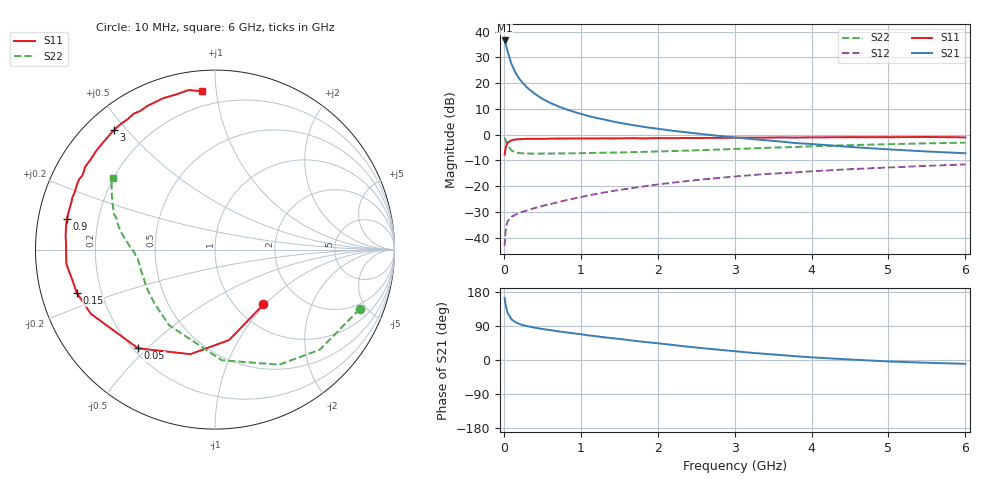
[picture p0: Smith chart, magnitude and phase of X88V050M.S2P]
! SIEMENS Small Signal Semiconductors
! BFP136W
! Si NPN RF Bipolar Junction Transistor in SOT343
! VCE = 8 V  IC = 50 mA
! Common Emitter S-Parameters:  September  1994
# GHz  S  MA  R  50
!  f  S11  S21  S12  S22
! GHz  MAG  ANG  MAG  ANG  MAG  ANG  MAG  ANG
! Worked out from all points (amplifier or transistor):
!   40 points, 10 MHz to 6 GHz, reference 50 ohm
!   highest |S21| = 36.6 dB at 10 MHz (marker M1)
!   |S21| within 3 dB of that: start of sweep to 38.22 MHz
!   unconditionally stable (mu >= 1): 786.2 MHz to 2.952 GHz
!   at 200 MHz: K = 0.52, MSG = 26.1 dB, |S12| = -30.4 dB
!   at 1.5 GHz: K = 1.11, MAG = 11.1 dB, |S12| = -21.5 dB
!   at 6 GHz: K = 0.96, MSG = 2.2 dB, |S12| = -11.6 dB
!   S11 on the Smith chart (normalised r, x): 10 MHz: 1.33, -0.98; 50 MHz: 0.22, -0.47; 150 MHz: 0.11, -0.15; 900 MHz: 0.09, +0.10; 3 GHz: 0.08, +0.46; 6 GHz: 0.11, +0.91
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0.01  0.4077 -48.5  67.69 163.9  0.0068 72.5  0.8718 -22.3
0.02  0.5099 -81.1  60.83 149.9  0.012 61.3  0.8076 -43.6
0.03  0.5984 -103.2  53.79 139.0  0.0162 53.5  0.7343 -60.8
0.05  0.6972 -127.9  40.62 124.1  0.0209 42.1  0.6177 -86.5
0.1  0.7786 -152.6  23.51 107.4  0.0253 33.9  0.4929 -121.3
0.15  0.8069 -162.6  16.19 99.8  0.0278 33.6  0.4521 -137.9
0.2  0.8126 -168.0  12.24 95.3  0.0301 33.4  0.4388 -147.4
0.25  0.8238 -172.0  9.888 92.0  0.0319 35.1  0.4332 -153.4
0.3  0.8316 -174.5  8.285 89.5  0.0336 36.7  0.4286 -157.6
0.4  0.8298 -179.2  6.249 85.3  0.0374 40.0  0.4279 -163.1
0.5  0.831 177.4  4.988 81.8  0.0411 42.4  0.4284 -166.7
0.6  0.8356 175.0  4.163 79.0  0.0446 44.5  0.4294 -169.0
0.7  0.8385 172.1  3.586 75.8  0.0484 47.2  0.4312 -170.6
0.9  0.8418 168.3  2.808 70.5  0.0567 49.7  0.4343 -173.4
1.1  0.8419 163.5  2.294 64.9  0.0657 51.8  0.4396 -175.0
1.5  0.8468 156.6  1.704 55.5  0.0843 53.7  0.4503 -178.0
2.2  0.8555 144.1  1.188 39.6  0.1167 51.7  0.4797 177.0
3  0.8722 130.3  0.885 23.2  0.1538 46.4  0.5265 170.3
3.2  0.8749 127.0  0.826 19.4  0.1623 44.8  0.5389 168.3
4.5  0.8915 108.8  0.577 1.3  0.213 34.5  0.6252 155.9
5.5  0.9011 99.4  0.471 -7.3  0.2472 26.3  0.6785 148.2
6  0.885 94.7  0.435 -10.1  0.2642 22.1  0.6977 144.9
